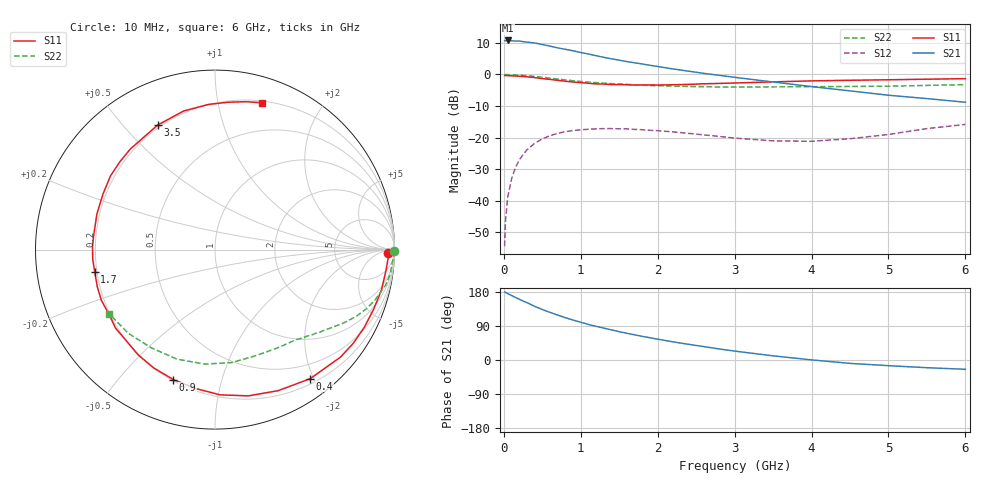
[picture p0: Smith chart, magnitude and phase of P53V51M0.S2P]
! SIEMENS Small Signal Semiconductors
! BFP183
! Si NPN RF Bipolar Junction Transistor in SOT143
! VCE = 3.5 V  IC = 1 mA
! Common Emitter S-Parameters:  March  1996
# GHz  S  MA  R  50
!  f  S11  S21  S12  S22
! GHz  MAG  ANG  MAG  ANG  MAG  ANG  MAG  ANG
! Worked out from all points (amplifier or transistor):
!   36 points, 10 MHz to 6 GHz, reference 50 ohm
!   highest |S21| = 10.8 dB at 50 MHz (marker M1)
!   |S21| within 3 dB of that: start of sweep to 841.3 MHz
!   unconditionally stable (mu >= 1): 2.473 GHz to end of sweep
!   at 250 MHz: K = 0.10, MSG = 17.9 dB, |S12| = -25.4 dB
!   at 1.4 GHz: K = 0.55, MSG = 11.1 dB, |S12| = -17.2 dB
!   at 6 GHz: K = 1.06, MAG = 2.0 dB, |S12| = -15.8 dB
!   S11 on the Smith chart (normalised r, x): 10 MHz: 41, -24; 400 MHz: 0.27, -1.95; 900 MHz: 0.21, -0.71; 1.7 GHz: 0.19, -0.09; 3.5 GHz: 0.19, +0.62; 6 GHz: 0.22, +1.35
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0.01  0.9646 -1.2  3.439 179.4  0.0019 85.3  0.9999 -0.5
0.02  0.9656 -2.9  3.427 178.6  0.0045 89.0  0.9962 -1.0
0.05  0.96 -6.8  3.463 175.1  0.0113 86.7  0.9954 -2.3
0.1  0.9544 -13.7  3.422 170.2  0.0221 81.5  0.989 -4.8
0.15  0.9443 -20.7  3.383 165.3  0.0334 77.4  0.9866 -7.3
0.2  0.9376 -27.5  3.395 160.4  0.044 73.3  0.9799 -9.5
0.4  0.8936 -53.6  3.159 141.7  0.0809 58.1  0.9324 -17.9
0.5  0.8611 -65.9  2.987 133.2  0.0954 50.9  0.9029 -21.6
0.6  0.8358 -77.2  2.82 125.7  0.1073 44.5  0.8745 -24.8
0.7  0.8097 -88.0  2.639 118.5  0.1167 38.9  0.8466 -27.5
0.9  0.7602 -107.8  2.375 105.4  0.1294 29.0  0.7966 -32.3
1.1  0.7262 -126.1  2.115 93.8  0.1357 20.9  0.7572 -36.3
1.3  0.7059 -141.7  1.869 84.1  0.1387 14.2  0.7284 -39.9
1.5  0.6933 -156.0  1.689 74.6  0.1378 8.8  0.7041 -43.1
1.7  0.6813 -169.6  1.532 66.5  0.1348 4.1  0.6843 -46.6
1.9  0.6828 178.6  1.4 58.7  0.1306 0.2  0.6691 -49.7
2.2  0.6873 163.2  1.224 47.9  0.1231 -3.9  0.6548 -54.9
2.8  0.7216 137.1  0.971 29.1  0.1044 -6.5  0.6345 -66.4
3.5  0.7636 114.8  0.76 11.0  0.0887 0.4  0.6361 -81.8
4.5  0.8097 92.5  0.55 -8.9  0.0959 19.6  0.646 -109.1
5.5  0.8421 78.1  0.415 -20.3  0.1388 26.8  0.6716 -136.0
6  0.8585 72.3  0.363 -24.5  0.1617 24.0  0.6896 -148.8
